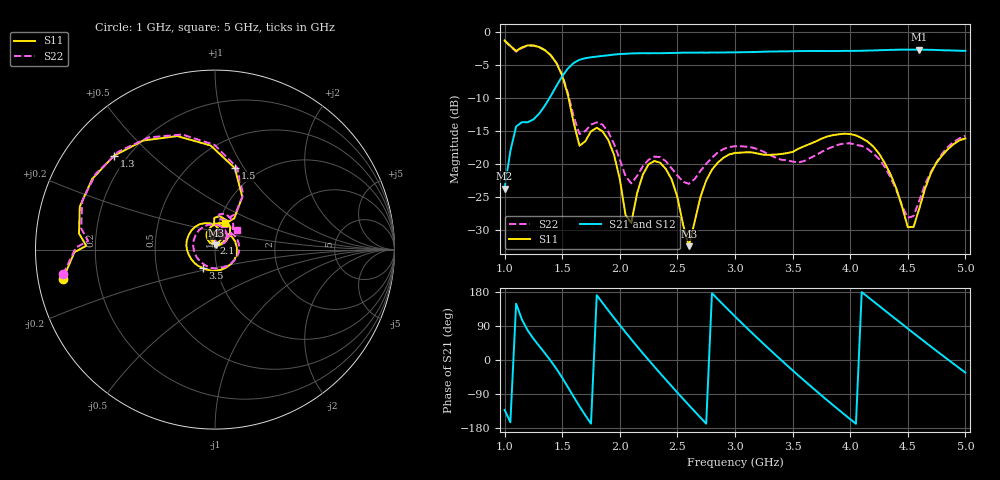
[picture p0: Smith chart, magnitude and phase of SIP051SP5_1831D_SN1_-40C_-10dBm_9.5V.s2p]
# GHz  S  dB  R  50
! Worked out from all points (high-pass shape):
!   81 points, 1 GHz to 5 GHz, reference 50 ohm
!   highest |S21| = -2.68 dB at 4.6 GHz (marker M1); lowest = -23.7 dB at 1 GHz (marker M2)
!   |S21| within 3 dB of the highest: 1.543 GHz to end of sweep
!   lowest |S11| = -32.4 dB at 2.6 GHz (marker M3), VSWR 1.05, Z = 50.5 + j2.34 ohm
!   |S11| at or under -10 dB: 1.555 GHz to end of sweep
!   |S22| runs from -28.1 to -1.3 dB; largest |S21 - S12| = 0.0017
!   S11 on the Smith chart (normalised r, x): 1 GHz: 0.08, -0.09; 1.3 GHz: 0.15, +0.38; 1.5 GHz: 0.78, +0.91; 2.1 GHz: 0.99, +0.07; 3.5 GHz: 0.85, -0.18; 5 GHz: 1.06, +0.32
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1  -1.30 -169.2  -23.71 -131.6  -23.72 -131.4  -1.33 -170.8
1.1  -2.88 178.3  -14.32 148.6  -14.30 148.7  -3.00 176.1
1.3  -2.29 137.2  -12.38 37.0  -12.37 37.1  -2.32 134.4
1.5  -6.61 76.3  -6.72 -46.9  -6.71 -46.9  -6.50 74.9
1.6  -13.78 58.4  -4.70 -97.3  -4.70 -97.3  -12.86 60.3
1.7  -16.57 92.1  -3.98 -145.7  -3.98 -145.7  -15.02 84.8
1.8  -14.52 82.1  -3.74 171.0  -3.73 171.0  -13.68 74.8
1.95  -18.62 44.9  -3.43 111.3  -3.44 111.3  -16.96 45.5
2.1  -28.92 98.9  -3.25 54.3  -3.25 54.3  -22.93 65.6
2.35  -19.80 70.3  -3.23 -35.0  -3.22 -34.9  -18.96 58.8
2.6  -32.44 75.5  -3.14 -119.3  -3.14 -119.3  -22.99 57.5
2.8  -20.86 82.1  -3.13 176.3  -3.12 176.3  -19.05 57.9
3  -18.33 21.5  -3.10 115.0  -3.08 115.0  -17.30 24.3
3.3  -18.61 -72.2  -2.98 27.9  -2.98 27.9  -18.61 -42.2
3.5  -18.17 -124.3  -2.92 -27.2  -2.92 -27.3  -19.63 -104.2
3.7  -16.60 -167.8  -2.90 -80.3  -2.90 -80.3  -18.67 -174.0
4.05  -15.66 120.2  -2.87 -168.4  -2.86 -168.4  -17.10 93.0
4.35  -21.56 64.5  -2.72 118.8  -2.74 118.8  -22.02 38.3
4.5  -29.56 80.5  -2.70 82.9  -2.69 83.0  -28.14 55.3
4.6  -26.75 126.3  -2.68 59.2  -2.69 59.2  -25.52 89.9
4.8  -18.67 108.7  -2.78 12.3  -2.78 12.4  -18.38 75.9
5  -16.13 69.8  -2.86 -33.3  -2.87 -33.4  -15.72 41.1
